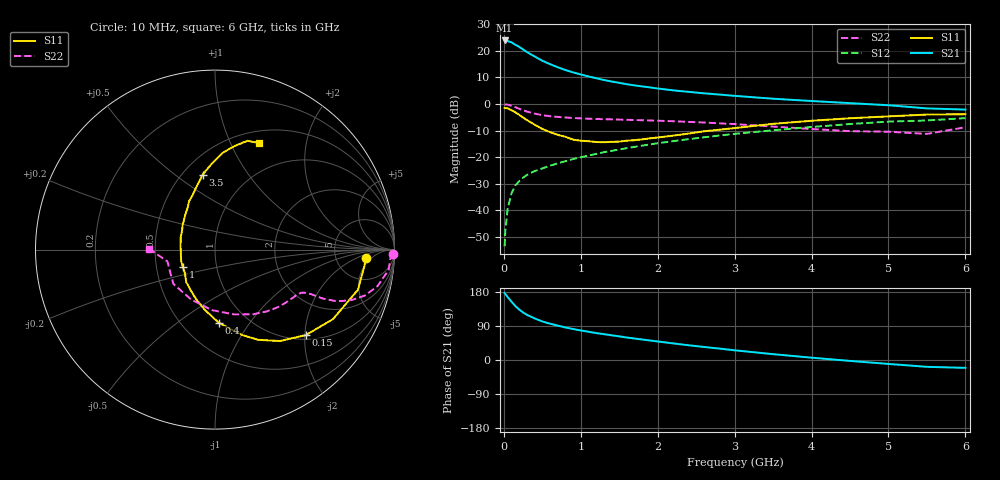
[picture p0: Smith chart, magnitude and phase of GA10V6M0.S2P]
! Infineon Technologies  Discrete & RF Semiconductors
! BF775
! Si NPN RF Bipolar Junction Transistor in SOT23
! VCE = 10 V  IC = 6 mA
! Common Emitter S-Parameters:  May  1996
# GHz  S  MA  R  50
!  f  S11  S21  S12  S22
! GHz  MAG  ANG  MAG  ANG  MAG  ANG  MAG  ANG
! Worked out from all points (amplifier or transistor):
!   36 points, 10 MHz to 6 GHz, reference 50 ohm
!   highest |S21| = 23.9 dB at 10 MHz (marker M1)
!   |S21| within 3 dB of that: start of sweep to 230.1 MHz
!   unconditionally stable (mu >= 1): 810.7 MHz to 2.907 GHz
!   at 250 MHz: K = 0.52, MSG = 24.1 dB, |S12| = -27.7 dB
!   at 1.4 GHz: K = 1.10, MAG = 11.2 dB, |S12| = -17.7 dB
!   at 6 GHz: K = 0.88, MSG = 1.6 dB, |S12| = -5.3 dB
!   S11 on the Smith chart (normalised r, x): 10 MHz: 11, -3; 150 MHz: 1.10, -2.03; 400 MHz: 0.74, -0.72; 1 GHz: 0.68, -0.14; 3.5 GHz: 0.62, +0.63; 6 GHz: 0.64, +1.29
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0.01  0.8423 -3.1  15.74 176.8  0.0021 91.2  0.9925 -1.3
0.02  0.8375 -6.3  15.44 174.0  0.0042 87.1  0.9789 -2.7
0.05  0.8273 -15.7  15.33 166.2  0.0108 78.9  0.9738 -6.7
0.1  0.763 -30.5  14.48 153.8  0.0208 75.2  0.9277 -12.7
0.15  0.6953 -43.2  13.08 142.2  0.0293 69.0  0.8726 -17.1
0.2  0.625 -54.6  11.92 133.1  0.0353 65.6  0.8144 -20.1
0.25  0.5574 -64.4  10.66 125.4  0.041 62.1  0.7621 -22.1
0.3  0.4993 -72.4  9.516 119.3  0.046 61.1  0.7217 -23.3
0.4  0.4072 -87.2  7.849 109.8  0.0544 59.6  0.6599 -24.4
0.5  0.3391 -99.9  6.542 101.7  0.0612 59.6  0.6155 -24.7
0.6  0.2955 -110.9  5.631 95.9  0.0688 60.1  0.5888 -24.9
0.7  0.2623 -121.5  4.934 90.6  0.0761 60.6  0.5714 -25.3
0.8  0.2417 -131.5  4.368 85.9  0.0838 60.5  0.5569 -25.6
1  0.2037 -151.6  3.596 78.0  0.0991 61.7  0.5364 -26.7
1.1  0.1993 -161.3  3.311 74.6  0.1072 61.8  0.5289 -27.8
1.3  0.1906 -178.5  2.836 68.2  0.1233 61.7  0.5173 -29.7
1.6  0.2037 159.5  2.355 59.3  0.1476 60.8  0.5037 -33.4
2.2  0.2535 131.1  1.809 43.8  0.1996 57.7  0.4743 -42.7
3.5  0.4233 99.4  1.258 15.4  0.3201 46.0  0.3759 -73.8
4.5  0.5391 85.7  1.038 -2.4  0.4194 34.3  0.3082 -115.5
5.5  0.6325 73.4  0.827 -18.0  0.4898 19.0  0.2735 -166.2
6  0.6419 67.6  0.785 -20.8  0.5419 14.8  0.3653 179.6
